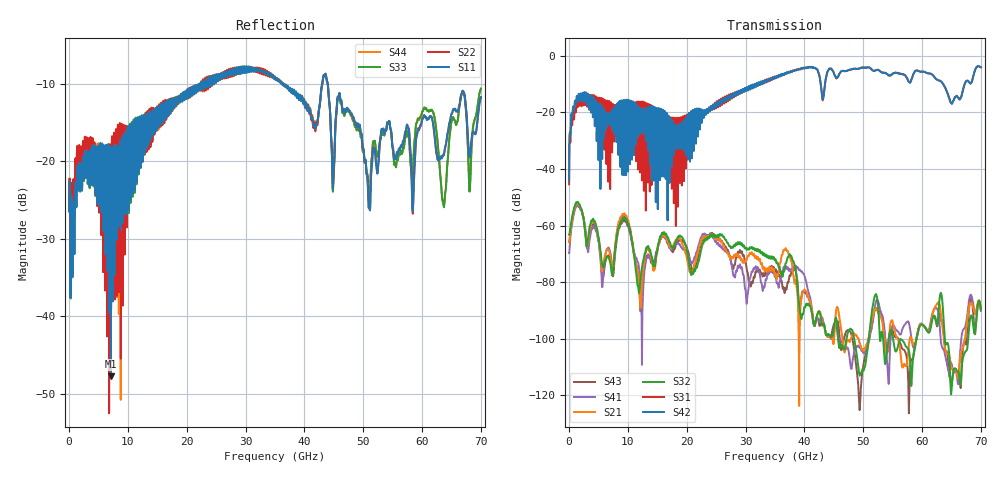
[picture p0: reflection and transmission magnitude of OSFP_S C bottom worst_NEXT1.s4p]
! AWR Design Environment (8415) Mon Jan 07 17:46:44 2019
! Document = 'OSFP Channel_S'
! nPorts: 4, nXvals: 7001
# HZ S DB R 50
!Freq DBS11 AngS11 DBS12 AngS12 DBS13 AngS13 DBS14 AngS14
!	DBS21 AngS21 DBS22 AngS22 DBS23 AngS23 DBS24 AngS24
!	DBS31 AngS31 DBS32 AngS32 DBS33 AngS33 DBS34 AngS34
!	DBS41 AngS41 DBS42 AngS42 DBS43 AngS43 DBS44 AngS44
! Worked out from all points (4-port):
!   7000 points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, 10 MHz to 70 GHz, reference 50 ohm
!   strongest paths, dB at 10 MHz, 17.51 GHz, 35.01 GHz, 52.51 GHz, 70 GHz:
!     S42: -44.0, -26.1, -7.4, -4.9, -4.0
!     S31: -45.4, -29.5, -7.4, -4.9, -4.0
!     S32: -63.3, -67.4, -72.2, -88.3, -89.5
!     S21: -65.8, -67.4, -77.2, -90.8, -89.4
!     S41: -69.8, -68.0, -78.0, -86.7, -89.9
!     S43: -65.8, -68.8, -75.8, -90.3, -90.1
!   lowest |S11| = -47.7 dB at 7.12 GHz (marker M1), VSWR 1.01, Z = 50.1 - j0.408 ohm
!   |S11| at or under -10 dB: start of sweep to 22.43 GHz; 36.33 GHz to 43.05 GHz (6.718 GHz wide, 16.9 % of centre); 43.97 GHz to end of sweep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
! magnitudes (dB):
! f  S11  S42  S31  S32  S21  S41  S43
! 10 MHz  -26.5  -44.0  -45.4  -63.3  -65.8  -69.8  -65.8
! 1.62 GHz  -22.0  -13.4  -15.0  -52.2  -52.6  -53.4  -52.9
! 7.12 GHz  -47.7  -24.7  -16.7  -74.4  -71.8  -70.5  -73.2
! 9.4 GHz  -19.3  -25.7  -22.5  -57.1  -55.7  -56.4  -57.9
! 12.14 GHz  -20.7  -19.5  -18.8  -79.0  -88.5  -80.2  -90.0
! 24.27 GHz  -10.0  -19.2  -18.5  -63.2  -63.1  -63.3  -62.6
! 70 GHz  -11.8  -4.0  -4.0  -89.5  -89.4  -89.9  -90.1
